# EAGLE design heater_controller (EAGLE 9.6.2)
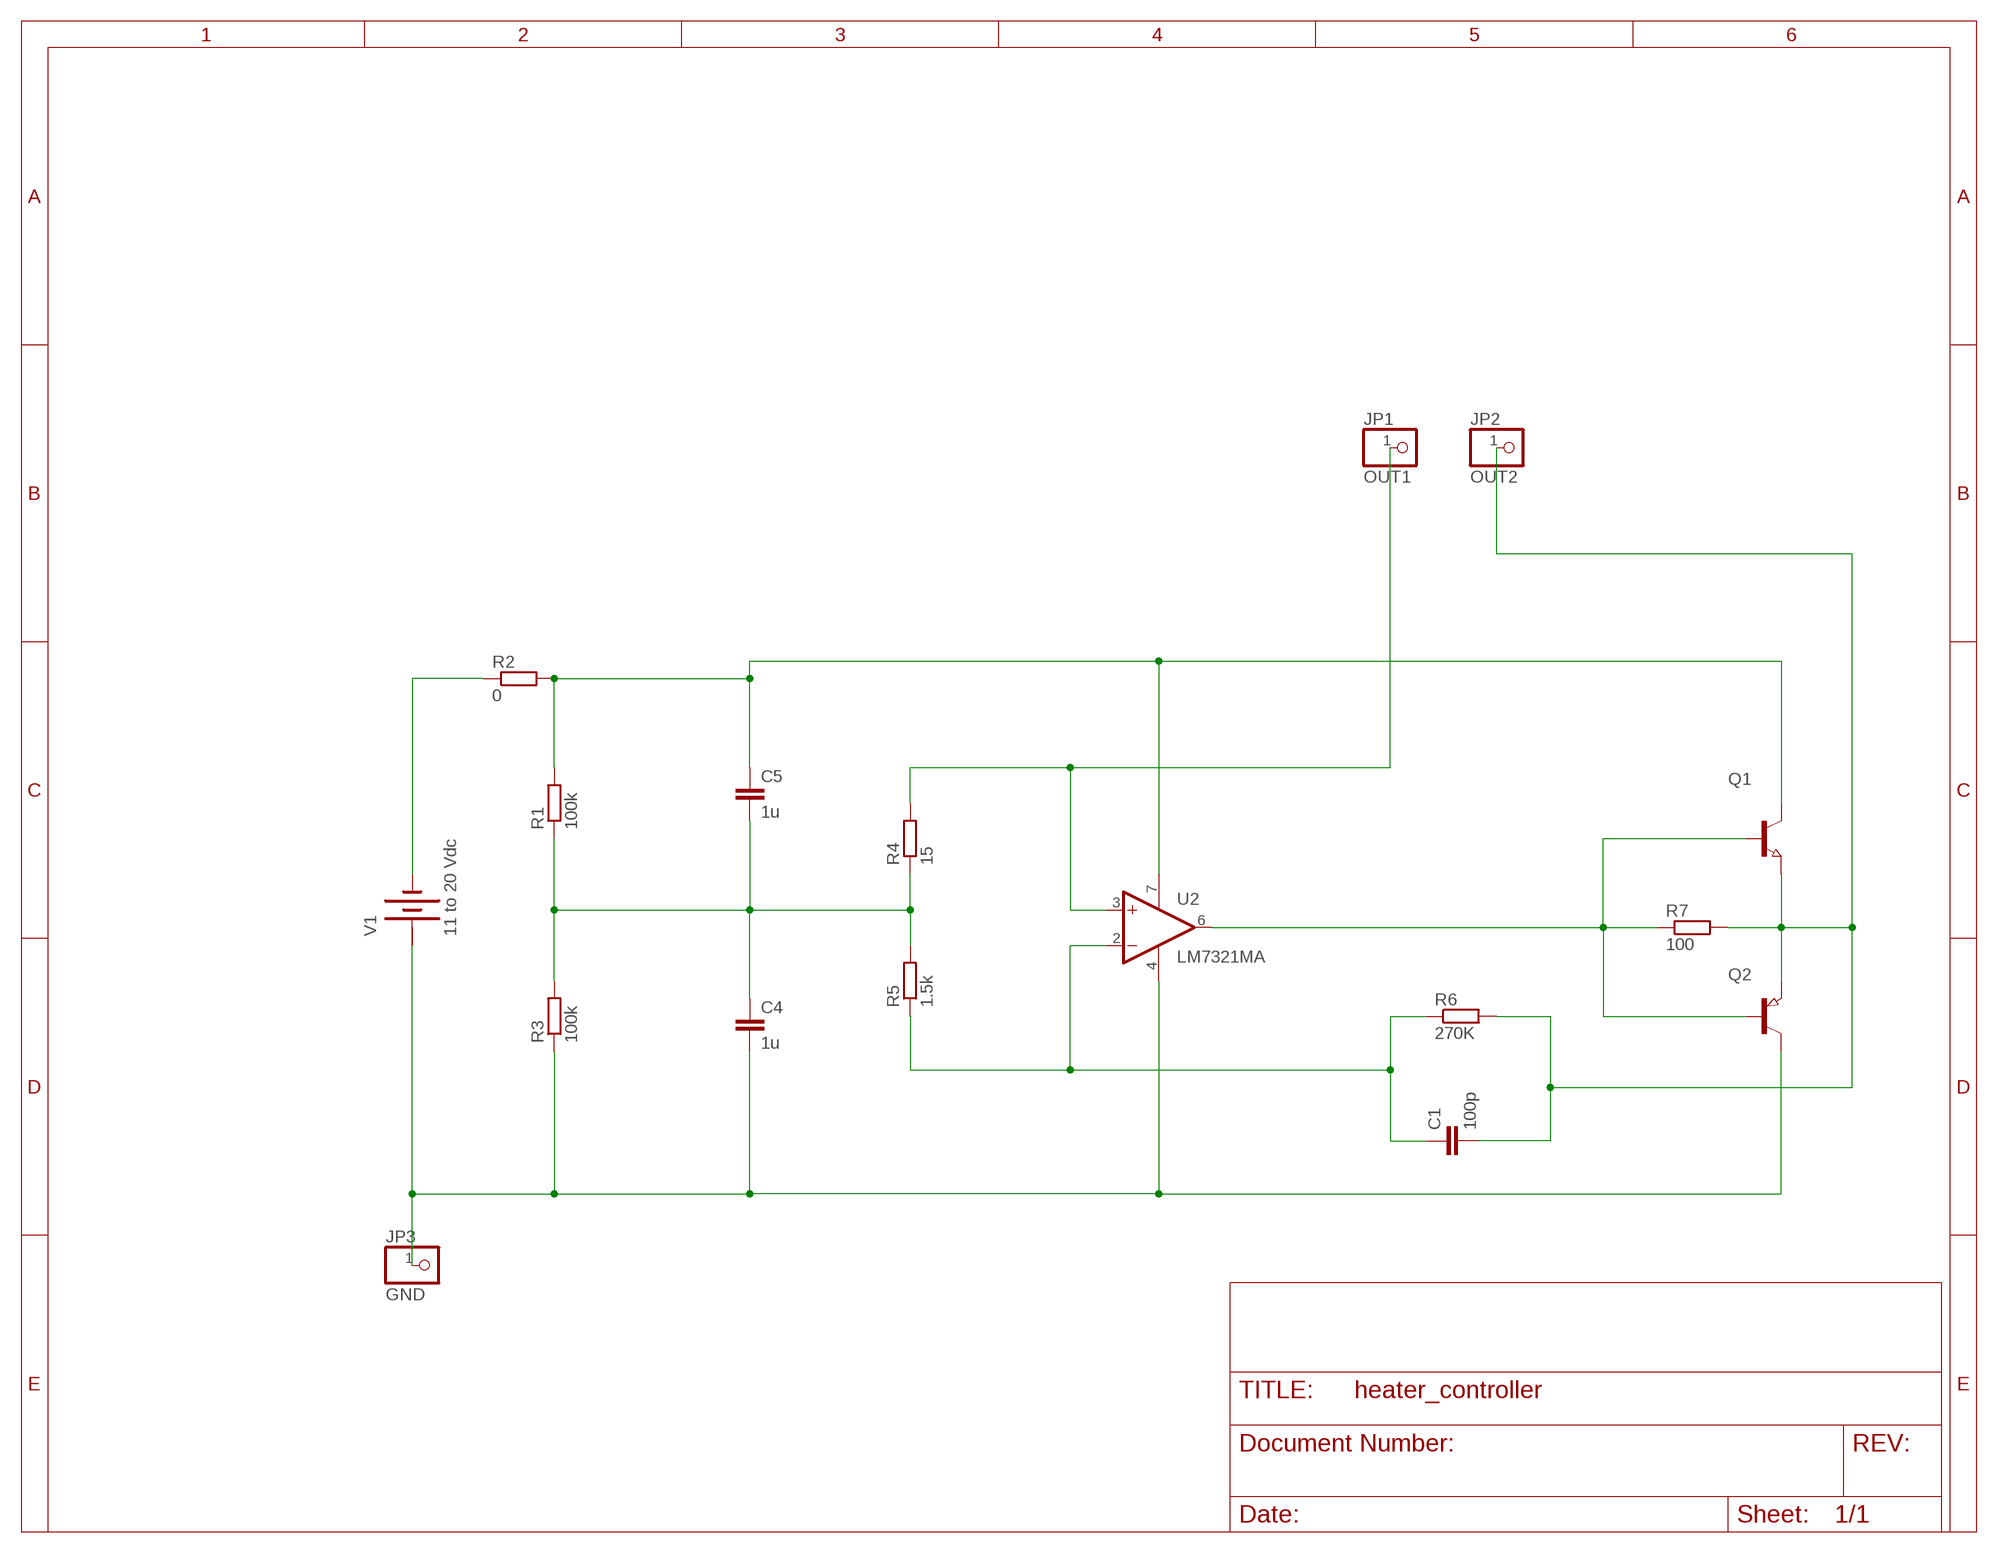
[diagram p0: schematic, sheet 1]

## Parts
C1  100p  C2,5-3  [C2.5-3]
C4  1u  C2,5-3  [C2.5-3]
C5  1u  C2,5-3  [C2.5-3]
JP1  OUT1  PINHD-1X1  [1X01]
JP2  OUT2  PINHD-1X1  [1X01]
JP3  GND  PINHD-1X1  [1X01]
Q1  NPN-TRANSISTOR_SOT23  [SOT23]
Q2  PNP-TRANSISTOR_SOT23W  [SOT23W]
R1  100k  R-EU_VMTA55  [VMTA55]
R2  0  R-EU_VMTA55  [VMTA55]
R3  100k  R-EU_VMTA55  [VMTA55]
R4  15  R-EU_VMTA55  [VMTA55]
R5  1.5k  R-EU_VMTA55  [VMTA55]
R6  270K  R-EU_VMTA55  [VMTA55]
R7  100  R-EU_VMTA55  [VMTA55]
U2  LM7321MA  OPA333D  [SO08]
V1  11 to 20 Vdc  BATTERY  [BATTERY]

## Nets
N$1: C4.2 JP3.1 Q2.3(C) R3.1 U2.4(V-) V1.+
N$2: C4.1 C5.2 R1.1 R3.2 R4.1 R5.2
N$3: C5.1 Q1.3(C) R1.2 R2.2 U2.7(V+)
N$4: JP1.1 R4.2 U2.3(+IN)
N$5: C1.1 R5.1 R6.1 U2.2(-IN)
N$6: R2.1 V1.-
N$7: Q1.1(B) Q2.1(B) R7.1 U2.6(OUT)
N$8: C1.2 JP2.1 Q1.2(E) Q2.2(E) R6.2 R7.2

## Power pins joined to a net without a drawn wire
+: V1.+@1(+)

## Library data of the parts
C1 C4 C5 = capacitor-wima:C: CAPACITOR
JP1-JP3 = pinhead:PINHD-1X1: PIN HEADER
Q1 = semicon-smd-ipc:NPN-TRANSISTOR_: NPN TRANSISTOR
Q2 = semicon-smd-ipc:PNP-TRANSISTOR_: PNP TRANSISTOR
R1-R7 = rcl:R-EU_: RESISTOR, European symbol; SPICEPREFIX: R
U2 = linear:OPA333: 1.8V, microPOWER CMOS OPERATIONAL AMPLIFIERS Zerø-Drift Series Source: Texas Instruments (Burr-Brown) .. U11 opa333 Operational Amp.pdf
V1 = special:BATTERY: BATTERY

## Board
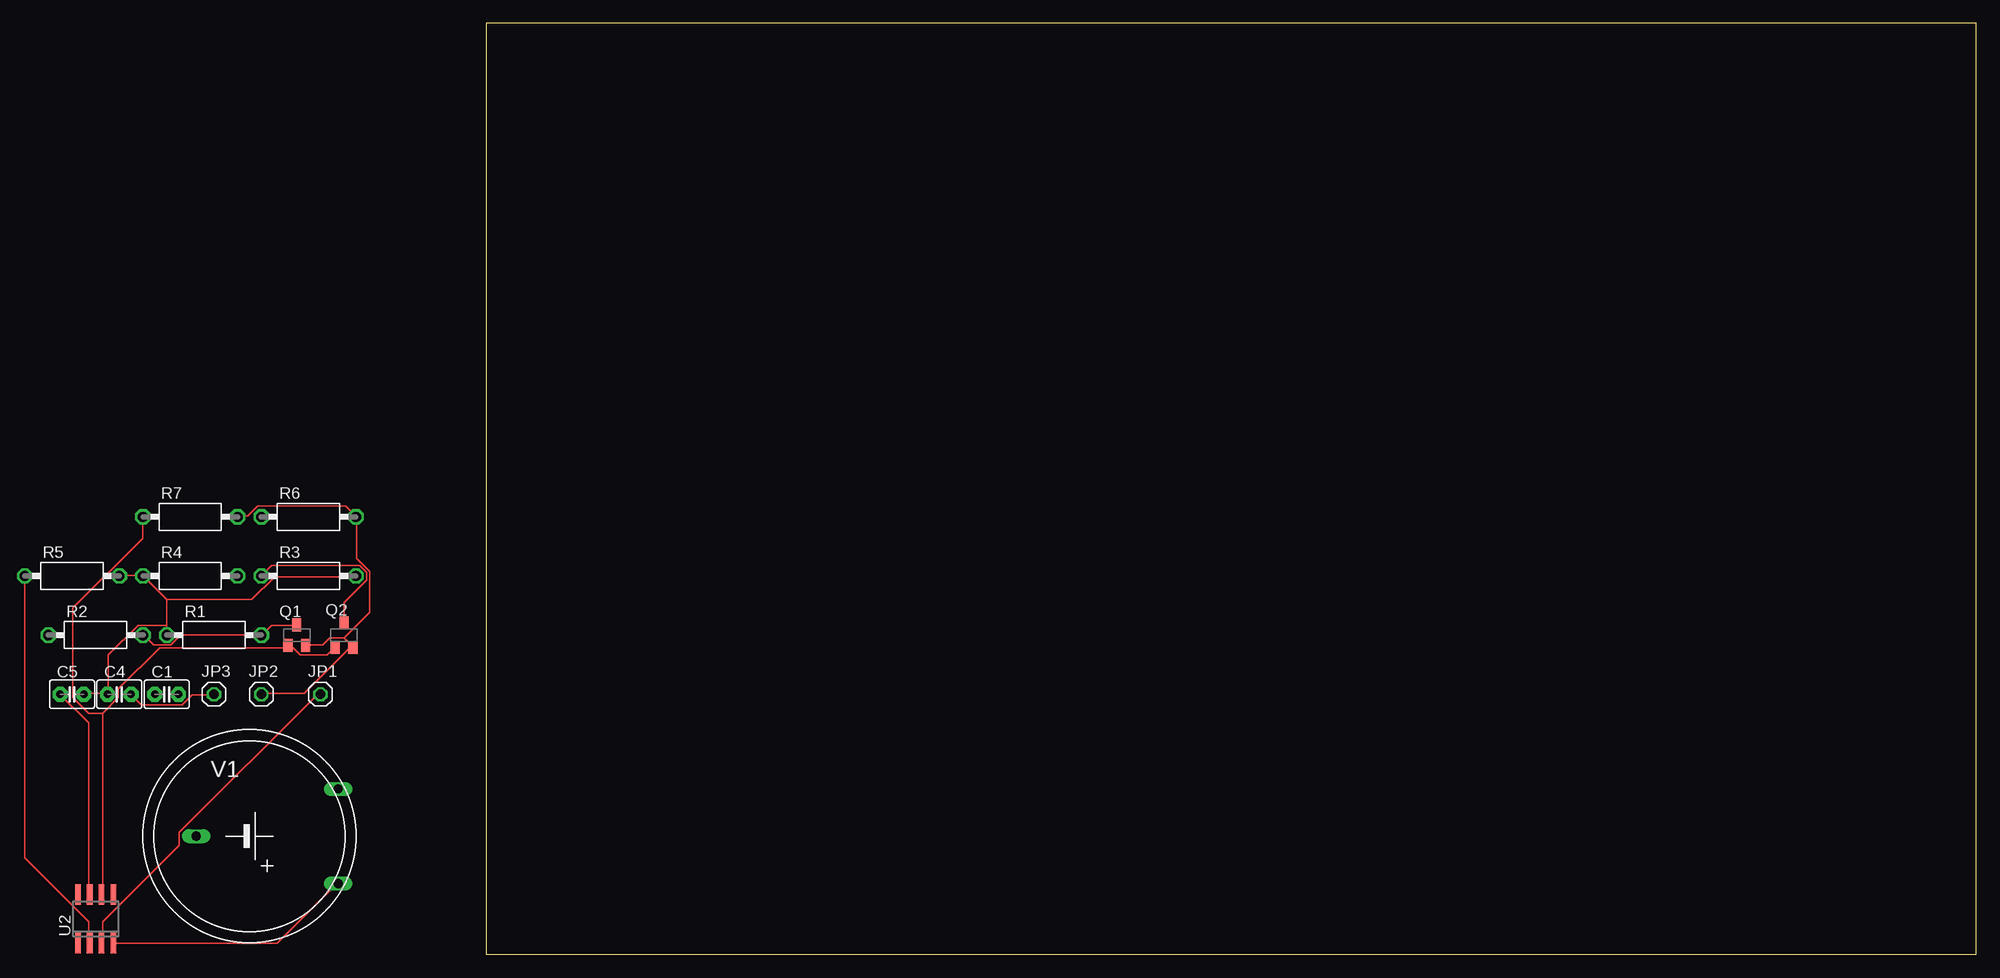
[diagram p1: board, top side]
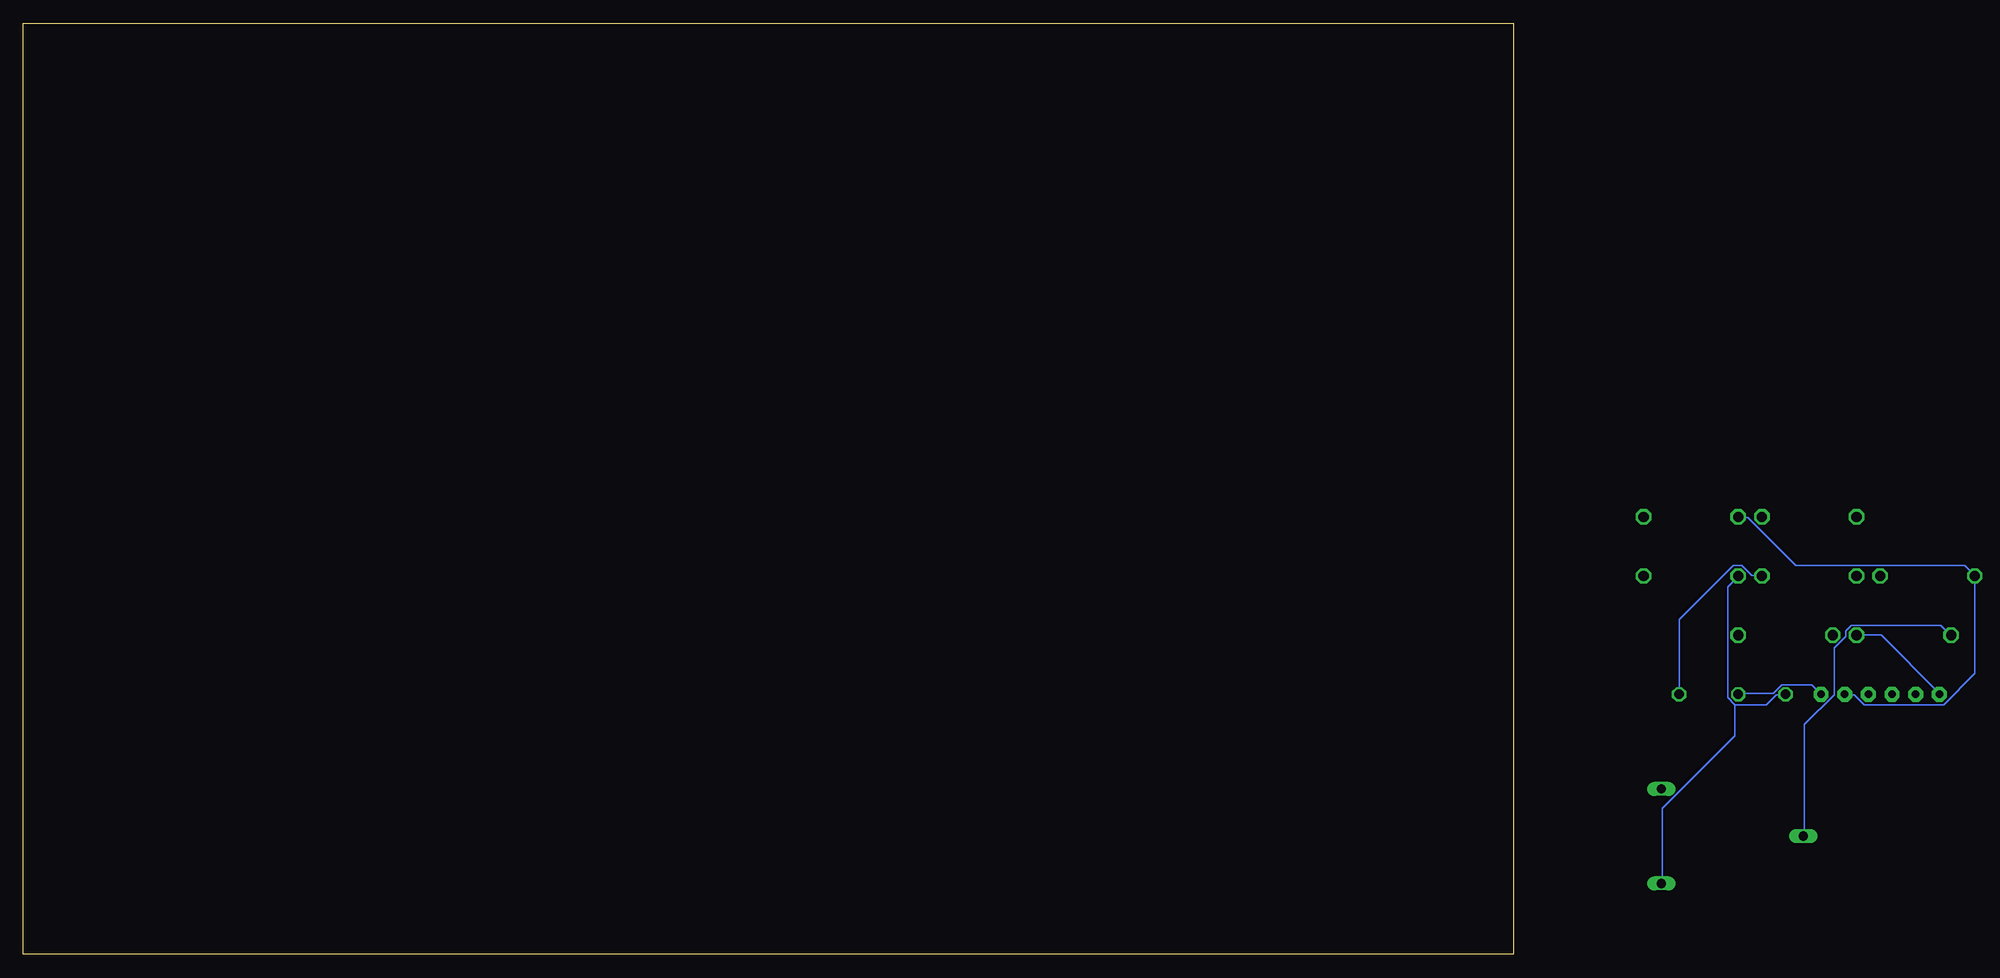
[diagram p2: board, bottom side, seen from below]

Size 160 x 100 mm. Coordinates in mm from the lower left corner, seen from the top.
Outline: 0,0 160,0 160,100 0,100 0,0
Copper layers (1*16): Top 0.035mm / dielectric 1.5mm / Bottom 0.035mm
Design rules "default": minimum track width 6mil, minimum drill 0.35mm, track to track 6mil, track to pad 6mil, pad to pad 6mil, via to via 6mil, smd to smd 6mil, copper to edge 40mil, drill to drill 6mil, minimum pad ring 10mil, minimum via ring 8mil, stop-mask expansion 4mil, vias tented up to drill 0mil, thermal gap 10mil

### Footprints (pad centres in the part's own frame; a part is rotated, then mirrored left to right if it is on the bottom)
C2.5-3 = drill 0.813 pad 1.6 octagon: 1 -1.27,0; 2 1.27,0
1X01 = drill 1.016 octagon: 1 0,0
SOT23 = smd 1 x 1.4: 1 -0.95,-1.1; 2 0.95,-1.1; 3 0,1.1
SOT23W = smd 1 x 1.4: 1 -0.95,-1.303; 2 0.95,-1.303; 3 0,1.303
VMTA55 = drill 1.1 octagon: 1 -5.08,0; 2 5.08,0
SO08 = smd 0.6 x 2.2: 1 -1.905,-2.6; 2 -0.635,-2.6; 3 0.635,-2.6; 4 1.905,-2.6; 5 1.905,2.6; 6 0.635,2.6; 7 -0.635,2.6; 8 -1.905,2.6
BATTERY = drill 1.016 long: + 9.525,-5.08; +@1 9.525,5.08; - -5.715,0

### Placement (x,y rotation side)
C1  -34.29,27.94 0 top  (outside the outline)
C4  -39.37,27.94 0 top  (outside the outline)
C5  -44.45,27.94 0 top  (outside the outline)
JP1  -17.78,27.94 0 top  (outside the outline)
JP2  -24.13,27.94 0 top  (outside the outline)
JP3  -29.21,27.94 0 top  (outside the outline)
Q1  -20.32,34.29 0 top  (outside the outline)
Q2  -15.24,34.29 0 top  (outside the outline)
R1  -29.21,34.29 0 top  (outside the outline)
R2  -41.91,34.29 0 top  (outside the outline)
R3  -19.05,40.64 0 top  (outside the outline)
R4  -31.75,40.64 0 top  (outside the outline)
R5  -44.45,40.64 0 top  (outside the outline)
R6  -19.05,46.99 0 top  (outside the outline)
R7  -31.75,46.99 0 top  (outside the outline)
U2  -41.91,3.81 0 top  (outside the outline)
V1  -25.4,12.7 0 top  (outside the outline)

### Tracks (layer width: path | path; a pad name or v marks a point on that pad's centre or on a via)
N$1
  Top 0.152: U2.4 -39.93,1.22 -22.4,1.22 -16,7.62 V1.+ | JP3.1 -29.26,27.89 -31.55,27.89 -32.61,26.82 -37.03,26.82 -38.1,27.89 C4.2 | Q2.3 -15.24,37.8 -12.8,40.23 -12.8,41 -13.56,41.76 -23.01,41.76 R3.1
  Bottom 0.152: -23.77,26.82 -27.13,26.82 -28.19,27.89 -29.11,27.89 JP3.1 | -23.77,26.82 -23.01,27.58 -23.01,39.47 -24.08,40.54 R3.1 | -23.77,26.82 -23.77,23.47 -16,15.7 -16,7.62 V1.+
N$2
  Top 0.152: C5.2 -43.13,28.04 -40.69,28.04 C4.1 -40.54,28.04 -40.54,32.16 -37.34,35.36 -34.29,35.36 | R5.2 -39.32,40.69 -36.88,40.69 R4.1 -34.29,38.1 | -34.29,38.1 -34.29,35.36 | -34.29,35.36 R1.1 | -34.29,38.1 -25.15,38.1 -22.71,40.54 -14.02,40.54 R3.2
N$3
  Top 0.152: Q1.3 -20.42,35.36 -23.01,35.36 -24.08,34.29 R1.2 -32.77,34.29 -33.83,33.22 -35.66,33.22 -36.73,34.29 R2.2 | U2.7 -42.67,6.55 -42.67,24.84 -45.72,27.89 C5.1
  Bottom 0.152: R2.2 -39.47,34.29 -45.72,28.04 C5.1
N$4
  Top 0.152: U2.3 -41.15,1.22 -41.15,3.5 -32.92,11.73 -32.92,13.11 -18.14,27.89 -17.83,27.89 JP1.1
  Bottom 0.152: R4.2 -26.67,40.69 -25.6,40.69 -24.54,41.76 -23.62,41.76 -17.83,35.97 -17.83,28.04 JP1.1
N$5
  Top 0.152: R5.1 -49.53,10.36 -42.67,3.5 -42.67,1.22 U2.2
  Bottom 0.152: C1.1 -35.66,27.89 -36.58,27.89 -37.64,26.82 -46.18,26.82 -49.53,30.18 R5.1 -49.53,40.69 -48.46,41.76 -30.33,41.76 -25.15,46.94 -24.23,46.94 R6.1
N$6
  Bottom 0.152: V1.- -31.24,12.8 -31.24,24.69 -34.44,27.89 -34.44,32.92 -35.66,34.14 -35.66,34.75 -36.27,35.36 -45.87,35.36 -46.94,34.29 R2.1
N$7
  Top 0.152: Q2.1 -16.31,32.92 -17.07,32.16 -19.96,32.16 -20.88,33.07 -21.18,33.07 Q1.1 -21.34,33.07 -21.49,32.92 -35.05,32.92 -39.47,28.5 -39.47,27.58 -41.15,25.91 | -41.15,25.91 -41.15,6.55 U2.6 | -41.15,25.91 -42.67,25.91 -44.35,27.58 -44.35,37.19 -36.88,44.65 -36.88,46.94 R7.1
N$8
  Top 0.152: R7.2 -26.67,47.09 -25.6,47.09 -24.54,48.16 -15.09,48.16 -14.02,47.09 R6.2 -13.87,46.94 -13.87,42.52 -12.5,41.15 -12.5,36.73 -15.24,33.98 | -15.24,33.98 -16.76,33.98 -17.53,33.22 -19.36,33.22 Q1.2 | -15.24,33.98 -14.33,33.07 Q2.2 -14.33,32.92 -14.63,32.92 -19.51,28.04 -24.08,28.04 JP2.1
  Bottom 0.152: C1.2 -32,28.96 -28.8,28.96 -27.89,28.04 -24.23,28.04 JP2.1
